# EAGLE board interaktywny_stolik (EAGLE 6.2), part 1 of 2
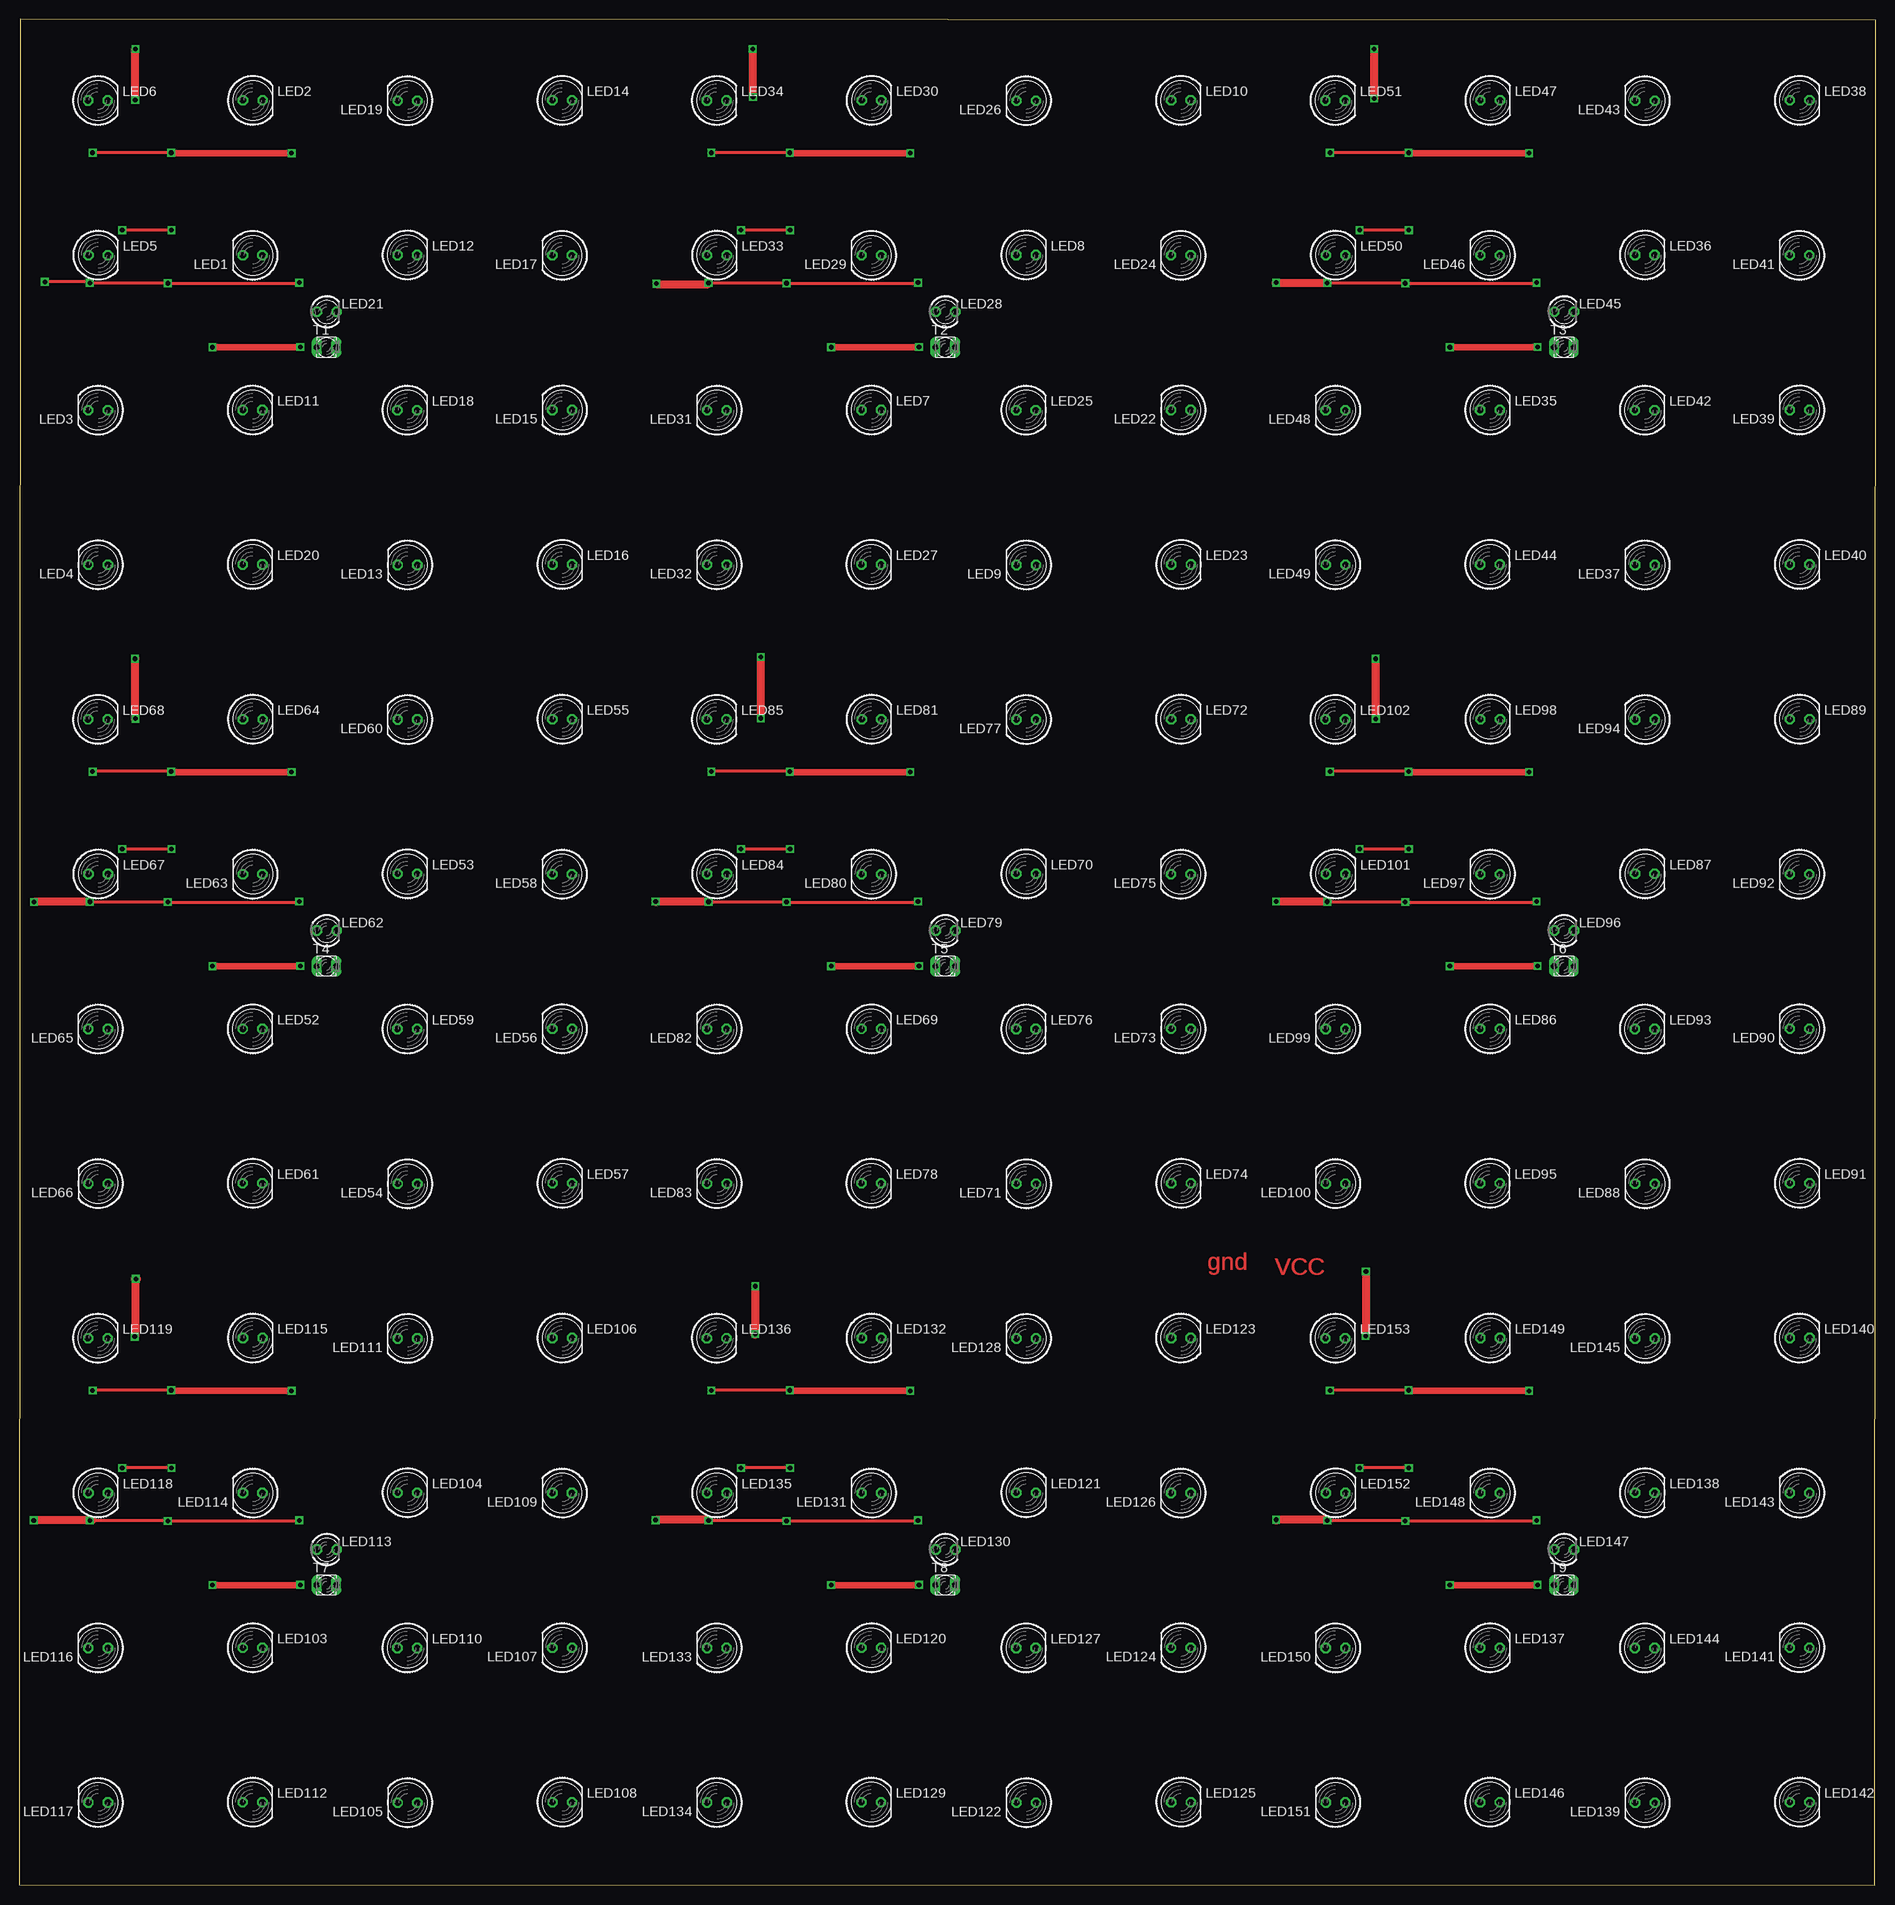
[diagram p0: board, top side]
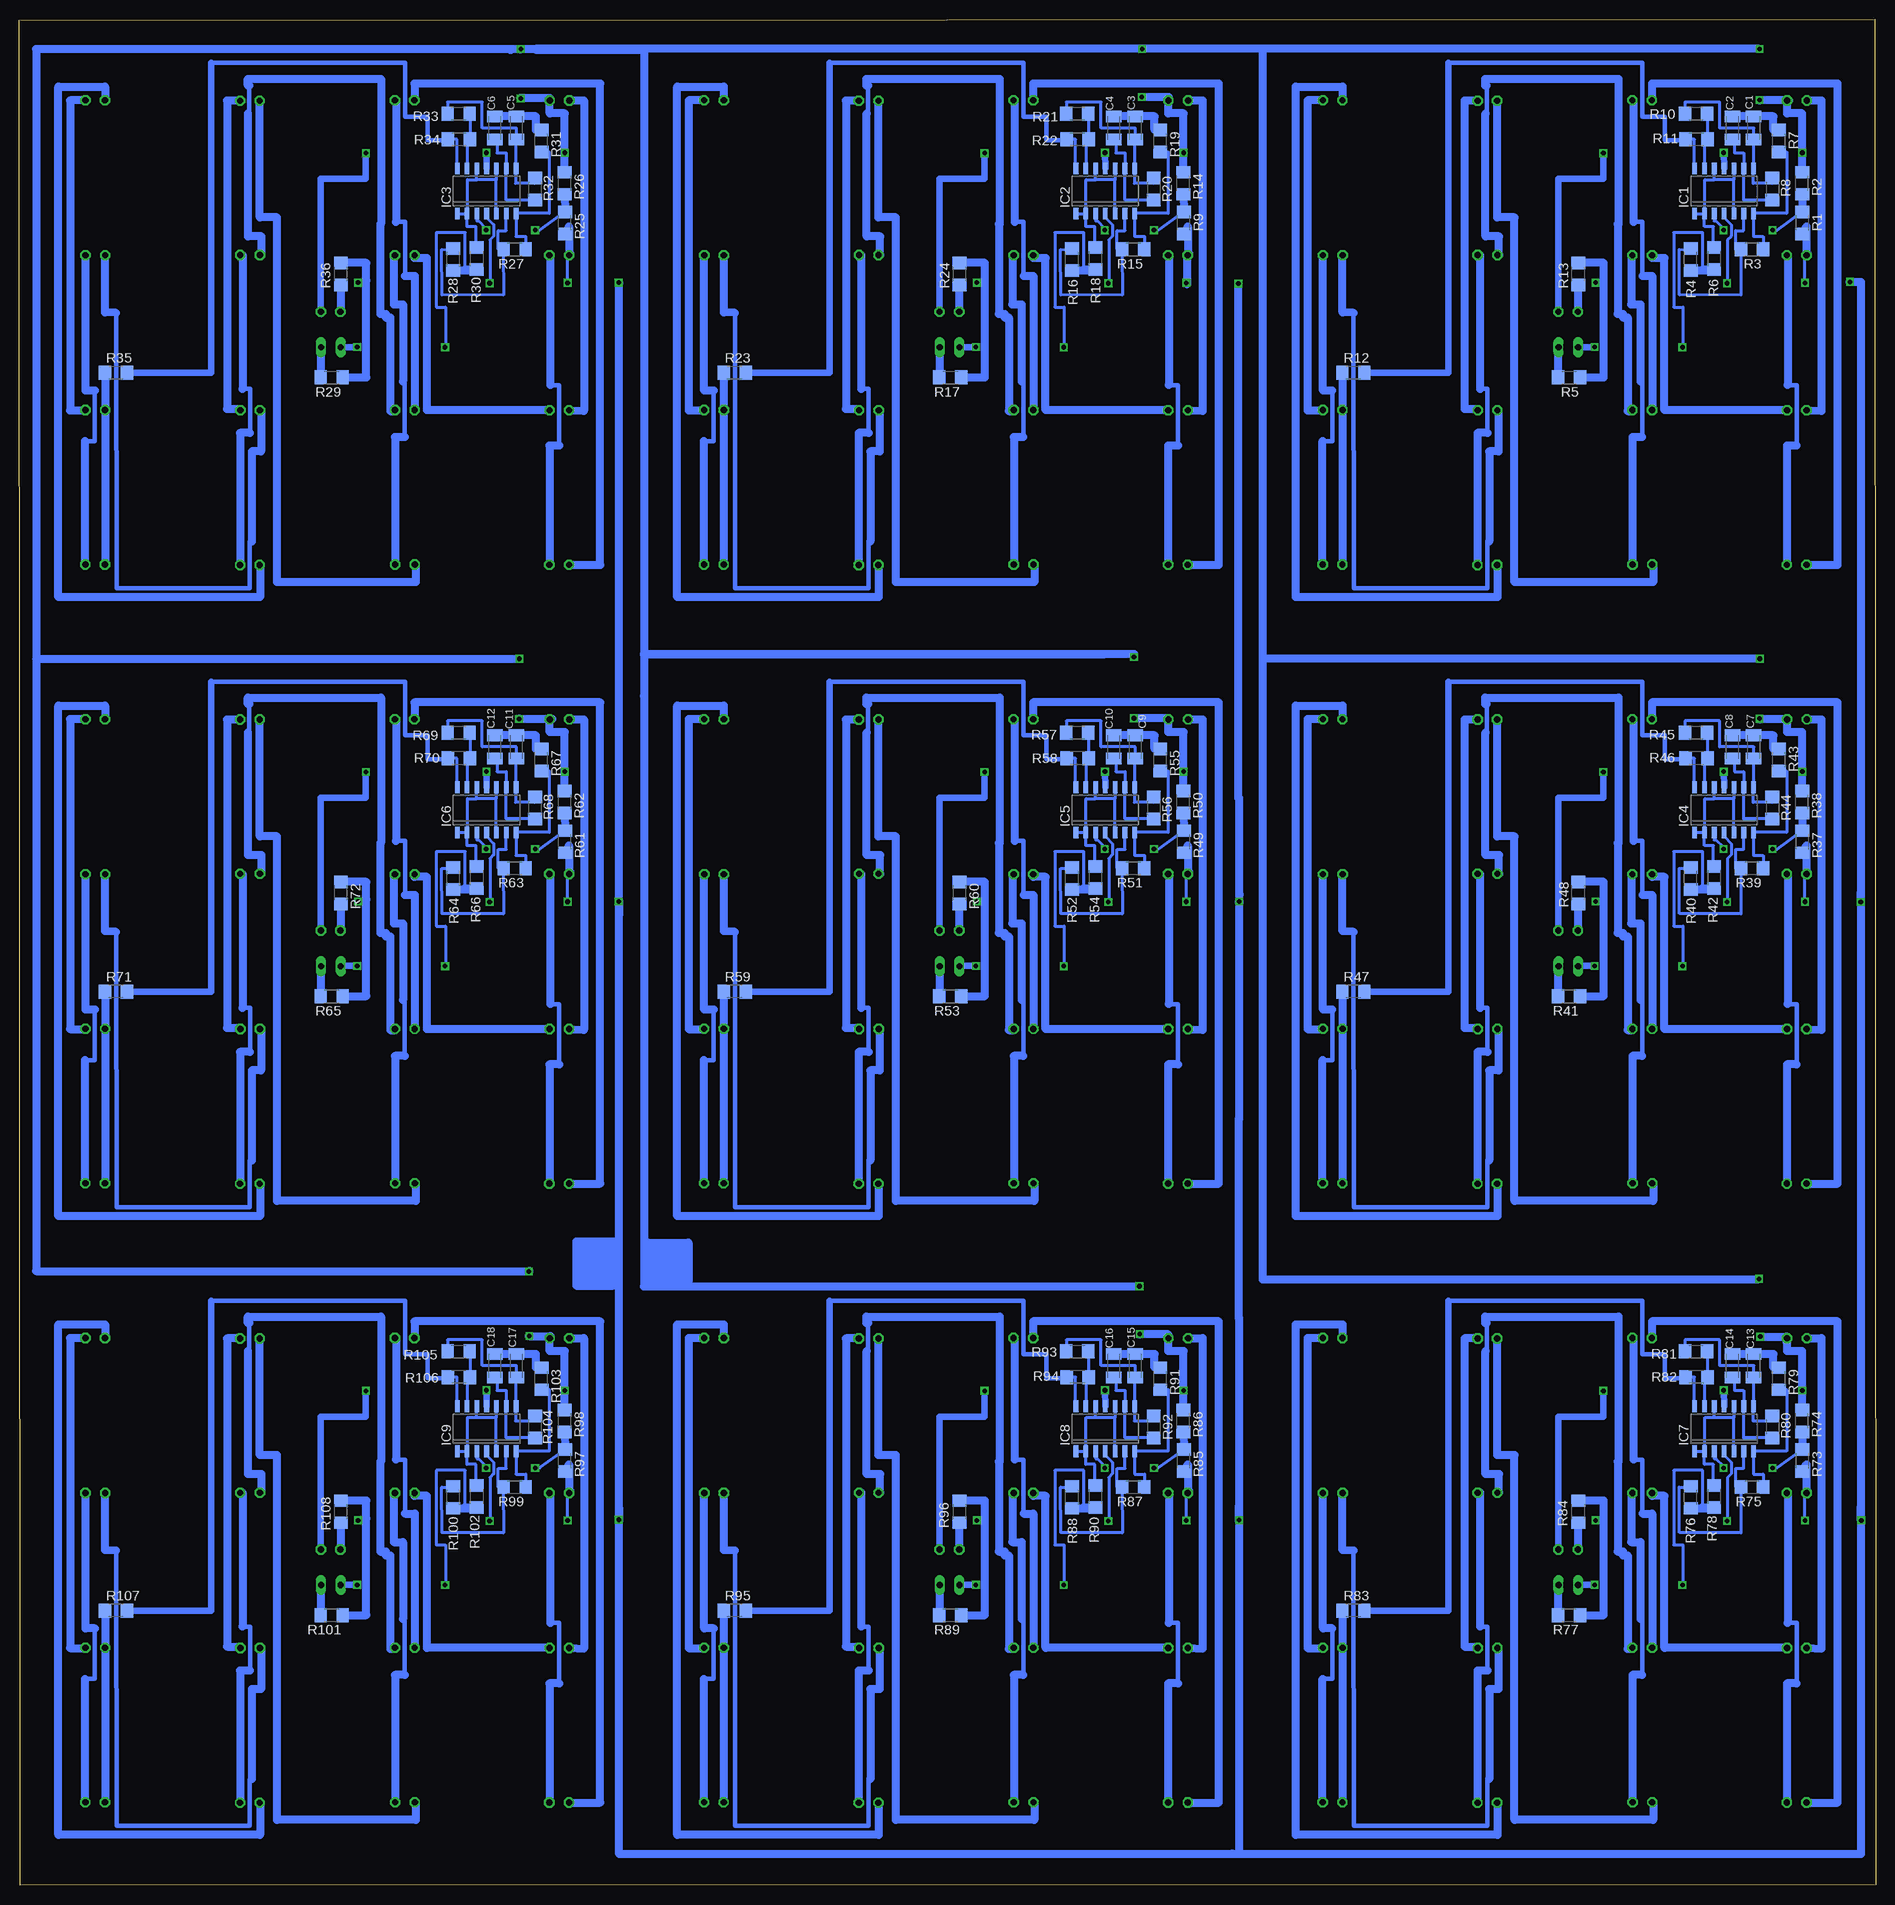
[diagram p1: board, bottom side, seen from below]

Size 240.01 x 241.21 mm. Coordinates in mm from the lower left corner, seen from the top.
Outline: 0,0.1 239.91,0 240.01,241.11 0.1,241.21 0,0.1
Copper layers (1*16): Top 0.035mm / dielectric 1.5mm / Bottom 0.035mm
Design rules: minimum track width 10mil, minimum drill 24mil, track to track 8mil, track to pad 8mil, pad to pad 8mil, via to via 8mil, smd to smd 8mil, copper to edge 40mil, drill to drill 8mil, minimum pad ring 10mil, minimum via ring 8mil, stop-mask expansion 4mil, vias tented up to drill 0mil, thermal gap 10mil

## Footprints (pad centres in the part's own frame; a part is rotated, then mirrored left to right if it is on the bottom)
C1206K = smd 1.5 x 2: 1 -1.5,0; 2 1.5,0
SO14 = smd 0.6 x 1.524: 1 -3.81,-2.935; 2 -2.54,-2.935; 3 -1.27,-2.935; 4 0,-2.935; 5 1.27,-2.935; 6 2.54,-2.935; 7 3.81,-2.935; 8 3.81,2.9; 9 2.54,2.9; 10 1.27,2.9; 11 0,2.9; 12 -1.27,2.9; 13 -2.54,2.9; 14 -3.81,2.9
LED5MM = drill 0.813 octagon: A -1.27,0; K 1.27,0
LED3MM = drill 0.813 octagon: A -1.27,0; K 1.27,0
R1206 = smd 1.6 x 1.803: 1 -1.422,0; 2 1.422,0
BPX81 = drill 0.813 long: C 1.27,0; E -1.27,0

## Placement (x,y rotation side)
C1  [C1206K]  15.75,227.16 270 bottom
C2  [C1206K]  18.52,227.16 270 bottom
C3  [C1206K]  95.75,227.16 270 bottom
C4  [C1206K]  98.52,227.16 270 bottom
C5  [C1206K]  175.75,227.16 270 bottom
C6  [C1206K]  178.52,227.16 270 bottom
C7  [C1206K]  15.75,147.16 270 bottom
C8  [C1206K]  18.52,147.16 270 bottom
C9  [C1206K]  95.75,147.16 270 bottom
C10  [C1206K]  98.52,147.16 270 bottom
C11  [C1206K]  175.75,147.16 270 bottom
C12  [C1206K]  178.52,147.16 270 bottom
C13  [C1206K]  15.75,67.16 270 bottom
C14  [C1206K]  18.52,67.16 270 bottom
C15  [C1206K]  95.75,67.16 270 bottom
C16  [C1206K]  98.52,67.16 270 bottom
C17  [C1206K]  175.75,67.16 270 bottom
C18  [C1206K]  178.52,67.16 270 bottom
IC1  LM324D  [SO14]  19.58,219.03 0 bottom
IC2  LM324D  [SO14]  99.58,219.03 0 bottom
IC3  LM324D  [SO14]  179.58,219.03 0 bottom
IC4  LM324D  [SO14]  19.58,139.03 0 bottom
IC5  LM324D  [SO14]  99.58,139.03 0 bottom
IC6  LM324D  [SO14]  179.58,139.03 0 bottom
IC7  LM324D  [SO14]  19.58,59.03 0 bottom
IC8  LM324D  [SO14]  99.58,59.03 0 bottom
IC9  LM324D  [SO14]  179.58,59.03 0 bottom
LED1  [LED5MM]  30.18,210.7 180 top
LED2  [LED5MM]  30.19,230.74 0 top
LED3  [LED5MM]  10.19,190.69 180 top
LED4  [LED5MM]  10.2,170.7 180 top
LED5  [LED5MM]  10.2,210.72 0 top
LED6  [LED5MM]  10.16,230.72 0 top
LED7  [LED5MM]  110.16,190.71 0 top
LED8  [LED5MM]  130.18,210.75 0 top
LED9  [LED5MM]  130.2,170.68 180 top
LED10  [LED5MM]  150.2,230.74 0 top
LED11  [LED5MM]  30.16,190.71 0 top
LED12  [LED5MM]  50.18,210.75 0 top
LED13  [LED5MM]  50.2,170.68 180 top
LED14  [LED5MM]  70.2,230.74 0 top
LED15  [LED5MM]  70.19,190.72 180 top
LED16  [LED5MM]  70.21,170.75 0 top
LED17  [LED5MM]  70.18,210.7 180 top
LED18  [LED5MM]  50.16,190.69 0 top
LED19  [LED5MM]  50.19,230.69 180 top
LED20  [LED5MM]  30.15,170.75 0 top
LED21  [LED3MM]  39.75,203.41 0 top
LED22  [LED5MM]  150.19,190.72 180 top
LED23  [LED5MM]  150.21,170.75 0 top
LED24  [LED5MM]  150.18,210.7 180 top
LED25  [LED5MM]  130.16,190.69 0 top
LED26  [LED5MM]  130.19,230.69 180 top
LED27  [LED5MM]  110.15,170.75 0 top
LED28  [LED3MM]  119.75,203.41 0 top
LED29  [LED5MM]  110.18,210.7 180 top
LED30  [LED5MM]  110.19,230.74 0 top
LED31  [LED5MM]  90.19,190.69 180 top
LED32  [LED5MM]  90.2,170.7 180 top
LED33  [LED5MM]  90.2,210.72 0 top
LED34  [LED5MM]  90.16,230.72 0 top
LED35  [LED5MM]  190.16,190.71 0 top
LED36  [LED5MM]  210.18,210.75 0 top
LED37  [LED5MM]  210.2,170.68 180 top
LED38  [LED5MM]  230.2,230.74 0 top
LED39  [LED5MM]  230.19,190.72 180 top
LED40  [LED5MM]  230.21,170.75 0 top
LED41  [LED5MM]  230.18,210.7 180 top
LED42  [LED5MM]  210.16,190.69 0 top
LED43  [LED5MM]  210.19,230.69 180 top
LED44  [LED5MM]  190.15,170.75 0 top
LED45  [LED3MM]  199.75,203.41 0 top
LED46  [LED5MM]  190.18,210.7 180 top
LED47  [LED5MM]  190.19,230.74 0 top
LED48  [LED5MM]  170.19,190.69 180 top
LED49  [LED5MM]  170.2,170.7 180 top
LED50  [LED5MM]  170.2,210.72 0 top
LED51  [LED5MM]  170.16,230.72 0 top
LED52  [LED5MM]  30.16,110.71 0 top
LED53  [LED5MM]  50.18,130.75 0 top
LED54  [LED5MM]  50.2,90.68 180 top
LED55  [LED5MM]  70.2,150.74 0 top
LED56  [LED5MM]  70.19,110.72 180 top
LED57  [LED5MM]  70.21,90.75 0 top
LED58  [LED5MM]  70.18,130.7 180 top
LED59  [LED5MM]  50.16,110.69 0 top
LED60  [LED5MM]  50.19,150.69 180 top
LED61  [LED5MM]  30.15,90.75 0 top
LED62  [LED3MM]  39.75,123.41 0 top
LED63  [LED5MM]  30.18,130.7 180 top
LED64  [LED5MM]  30.19,150.74 0 top
LED65  [LED5MM]  10.19,110.69 180 top
LED66  [LED5MM]  10.2,90.7 180 top
LED67  [LED5MM]  10.2,130.72 0 top
LED68  [LED5MM]  10.16,150.72 0 top
LED69  [LED5MM]  110.16,110.71 0 top
LED70  [LED5MM]  130.18,130.75 0 top
LED71  [LED5MM]  130.2,90.68 180 top
LED72  [LED5MM]  150.2,150.74 0 top
LED73  [LED5MM]  150.19,110.72 180 top
LED74  [LED5MM]  150.21,90.75 0 top
LED75  [LED5MM]  150.18,130.7 180 top
LED76  [LED5MM]  130.16,110.69 0 top
LED77  [LED5MM]  130.19,150.69 180 top
LED78  [LED5MM]  110.15,90.75 0 top
LED79  [LED3MM]  119.75,123.41 0 top
LED80  [LED5MM]  110.18,130.7 180 top
LED81  [LED5MM]  110.19,150.74 0 top
LED82  [LED5MM]  90.19,110.69 180 top
LED83  [LED5MM]  90.2,90.7 180 top
LED84  [LED5MM]  90.2,130.72 0 top
LED85  [LED5MM]  90.16,150.72 0 top
LED86  [LED5MM]  190.16,110.71 0 top
LED87  [LED5MM]  210.18,130.75 0 top
LED88  [LED5MM]  210.2,90.68 180 top
LED89  [LED5MM]  230.2,150.74 0 top
LED90  [LED5MM]  230.19,110.72 180 top
LED91  [LED5MM]  230.21,90.75 0 top
LED92  [LED5MM]  230.18,130.7 180 top
LED93  [LED5MM]  210.16,110.69 0 top
LED94  [LED5MM]  210.19,150.69 180 top
LED95  [LED5MM]  190.15,90.75 0 top
LED96  [LED3MM]  199.75,123.41 0 top
LED97  [LED5MM]  190.18,130.7 180 top
LED98  [LED5MM]  190.19,150.74 0 top
LED99  [LED5MM]  170.19,110.69 180 top
LED100  [LED5MM]  170.2,90.7 180 top
LED101  [LED5MM]  170.2,130.72 0 top
LED102  [LED5MM]  170.16,150.72 0 top
LED103  [LED5MM]  30.16,30.71 0 top
LED104  [LED5MM]  50.18,50.75 0 top
LED105  [LED5MM]  50.2,10.68 180 top
LED106  [LED5MM]  70.2,70.74 0 top
LED107  [LED5MM]  70.19,30.72 180 top
LED108  [LED5MM]  70.21,10.75 0 top
LED109  [LED5MM]  70.18,50.7 180 top
LED110  [LED5MM]  50.16,30.69 0 top
LED111  [LED5MM]  50.19,70.69 180 top
LED112  [LED5MM]  30.15,10.75 0 top
LED113  [LED3MM]  39.75,43.41 0 top
LED114  [LED5MM]  30.18,50.7 180 top
LED115  [LED5MM]  30.19,70.74 0 top
LED116  [LED5MM]  10.19,30.69 180 top
LED117  [LED5MM]  10.2,10.7 180 top
LED118  [LED5MM]  10.2,50.72 0 top
LED119  [LED5MM]  10.16,70.72 0 top
LED120  [LED5MM]  110.16,30.71 0 top
LED121  [LED5MM]  130.18,50.75 0 top
LED122  [LED5MM]  130.2,10.68 180 top
LED123  [LED5MM]  150.2,70.74 0 top
LED124  [LED5MM]  150.19,30.72 180 top
LED125  [LED5MM]  150.21,10.75 0 top
LED126  [LED5MM]  150.18,50.7 180 top
LED127  [LED5MM]  130.16,30.69 0 top
LED128  [LED5MM]  130.19,70.69 180 top
LED129  [LED5MM]  110.15,10.75 0 top
LED130  [LED3MM]  119.75,43.41 0 top
LED131  [LED5MM]  110.18,50.7 180 top
LED132  [LED5MM]  110.19,70.74 0 top
LED133  [LED5MM]  90.19,30.69 180 top
LED134  [LED5MM]  90.2,10.7 180 top
LED135  [LED5MM]  90.2,50.72 0 top
LED136  [LED5MM]  90.16,70.72 0 top
LED137  [LED5MM]  190.16,30.71 0 top
LED138  [LED5MM]  210.18,50.75 0 top
LED139  [LED5MM]  210.2,10.68 180 top
LED140  [LED5MM]  230.2,70.74 0 top
LED141  [LED5MM]  230.19,30.72 180 top
LED142  [LED5MM]  230.21,10.75 0 top
LED143  [LED5MM]  230.18,50.7 180 top
LED144  [LED5MM]  210.16,30.69 0 top
LED145  [LED5MM]  210.19,70.69 180 top
LED146  [LED5MM]  190.15,10.75 0 top
LED147  [LED3MM]  199.75,43.41 0 top
LED148  [LED5MM]  190.18,50.7 180 top
LED149  [LED5MM]  190.19,70.74 0 top
LED150  [LED5MM]  170.19,30.69 180 top
LED151  [LED5MM]  170.2,10.7 180 top
LED152  [LED5MM]  170.2,50.72 0 top
LED153  [LED5MM]  170.16,70.72 0 top
R1  [R1206]  9.45,214.89 270 bottom
R2  [R1206]  9.5,220.03 270 bottom
R3  [R1206]  15.98,211.49 180 bottom
R4  [R1206]  23.9,210.17 270 bottom
R5  [R1206]  39.62,194.93 180 bottom
R6  [R1206]  20.88,210.27 90 bottom
R7  [R1206]  12.5,225.49 270 bottom
R8  [R1206]  13.33,219.26 90 bottom
R9  [R1206]  89.45,214.89 270 bottom
R10  [R1206]  23.22,229.02 180 bottom
R11  [R1206]  23.16,225.69 0 bottom
R12  [R1206]  67.51,195.51 0 bottom
R13  [R1206]  38.43,208.29 270 bottom
R14  [R1206]  89.5,220.03 270 bottom
R15  [R1206]  95.98,211.49 180 bottom
R16  [R1206]  103.9,210.17 270 bottom
R17  [R1206]  119.62,194.93 180 bottom
R18  [R1206]  100.88,210.27 90 bottom
R19  [R1206]  92.5,225.49 270 bottom
R20  [R1206]  93.33,219.26 90 bottom
R21  [R1206]  103.22,229.02 180 bottom
R22  [R1206]  103.16,225.69 0 bottom
R23  [R1206]  147.51,195.51 0 bottom
R24  [R1206]  118.43,208.29 270 bottom
R25  [R1206]  169.45,214.89 270 bottom
R26  [R1206]  169.5,220.03 270 bottom
R27  [R1206]  175.98,211.49 180 bottom
R28  [R1206]  183.9,210.17 270 bottom
R29  [R1206]  199.62,194.93 180 bottom
R30  [R1206]  180.88,210.27 90 bottom
R31  [R1206]  172.5,225.49 270 bottom
R32  [R1206]  173.34,219.26 90 bottom
R33  [R1206]  183.22,229.02 180 bottom
R34  [R1206]  183.16,225.69 0 bottom
R35  [R1206]  227.51,195.51 0 bottom
R36  [R1206]  198.43,208.29 270 bottom
R37  [R1206]  9.45,134.89 270 bottom
R38  [R1206]  9.5,140.03 270 bottom
R39  [R1206]  15.98,131.49 180 bottom
R40  [R1206]  23.9,130.17 270 bottom
R41  [R1206]  39.62,114.93 180 bottom
R42  [R1206]  20.88,130.27 90 bottom
R43  [R1206]  12.5,145.49 270 bottom
R44  [R1206]  13.33,139.26 90 bottom
R45  [R1206]  23.22,149.02 180 bottom
R46  [R1206]  23.16,145.69 0 bottom
R47  [R1206]  67.51,115.51 0 bottom
R48  [R1206]  38.43,128.29 270 bottom
R49  [R1206]  89.45,134.89 270 bottom
R50  [R1206]  89.5,140.03 270 bottom
R51  [R1206]  95.98,131.49 180 bottom
R52  [R1206]  103.9,130.17 270 bottom
R53  [R1206]  119.62,114.93 180 bottom
R54  [R1206]  100.88,130.27 90 bottom
R55  [R1206]  92.5,145.49 270 bottom
R56  [R1206]  93.33,139.26 90 bottom
R57  [R1206]  103.22,149.02 180 bottom
R58  [R1206]  103.16,145.69 0 bottom
R59  [R1206]  147.51,115.51 0 bottom
R60  [R1206]  118.43,128.29 270 bottom
R61  [R1206]  169.45,134.89 270 bottom
R62  [R1206]  169.5,140.03 270 bottom
R63  [R1206]  175.98,131.49 180 bottom
R64  [R1206]  183.9,130.17 270 bottom
R65  [R1206]  199.62,114.93 180 bottom
R66  [R1206]  180.88,130.27 90 bottom
R67  [R1206]  172.5,145.49 270 bottom
R68  [R1206]  173.34,139.26 90 bottom
R69  [R1206]  183.22,149.02 180 bottom
R70  [R1206]  183.16,145.69 0 bottom
R71  [R1206]  227.51,115.51 0 bottom
R72  [R1206]  198.43,128.29 270 bottom
R73  [R1206]  9.45,54.89 270 bottom
R74  [R1206]  9.5,60.03 270 bottom
R75  [R1206]  15.98,51.49 180 bottom
R76  [R1206]  23.9,50.17 270 bottom
R77  [R1206]  39.62,34.93 180 bottom
R78  [R1206]  20.88,50.27 90 bottom
R79  [R1206]  12.5,65.49 270 bottom
R80  [R1206]  13.33,59.26 90 bottom
R81  [R1206]  23.22,69.02 180 bottom
R82  [R1206]  23.16,65.69 0 bottom
R83  [R1206]  67.51,35.51 0 bottom
R84  [R1206]  38.43,48.29 270 bottom
R85  [R1206]  89.45,54.89 270 bottom
R86  [R1206]  89.5,60.03 270 bottom
R87  [R1206]  95.98,51.49 180 bottom
R88  [R1206]  103.9,50.17 270 bottom
R89  [R1206]  119.62,34.93 180 bottom
R90  [R1206]  100.88,50.27 90 bottom
R91  [R1206]  92.5,65.49 270 bottom
R92  [R1206]  93.33,59.26 90 bottom
R93  [R1206]  103.22,69.02 180 bottom
R94  [R1206]  103.16,65.69 0 bottom
R95  [R1206]  147.51,35.51 0 bottom
R96  [R1206]  118.43,48.29 270 bottom
R97  [R1206]  169.45,54.89 270 bottom
R98  [R1206]  169.5,60.03 270 bottom
R99  [R1206]  175.98,51.49 180 bottom
R100  [R1206]  183.9,50.17 270 bottom
R101  [R1206]  199.62,34.93 180 bottom
R102  [R1206]  180.88,50.27 90 bottom
R103  [R1206]  172.5,65.49 270 bottom
R104  [R1206]  173.34,59.26 90 bottom
R105  [R1206]  183.22,69.02 180 bottom
R106  [R1206]  183.16,65.69 0 bottom
R107  [R1206]  227.51,35.51 0 bottom
R108  [R1206]  198.43,48.29 270 bottom
T1  BPX81  [BPX81]  39.73,198.82 0 top
T2  BPX81  [BPX81]  119.73,198.82 0 top
T3  BPX81  [BPX81]  199.73,198.82 0 top
T4  BPX81  [BPX81]  39.73,118.82 0 top
T5  BPX81  [BPX81]  119.73,118.82 0 top
T6  BPX81  [BPX81]  199.73,118.82 0 top
T7  BPX81  [BPX81]  39.73,38.82 0 top
T8  BPX81  [BPX81]  119.73,38.82 0 top
T9  BPX81  [BPX81]  199.73,38.82 0 top

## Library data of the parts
C1-C18 R1-R108 = rcl
IC1-IC9 = linear
LED1-LED153 = led
T1-T9 = opto-trans-siemens; OC_FARNELL: unknown; OC_NEWARK: unknown

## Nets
0V: IC1.1 IC1.2 IC1.5 IC1.10 IC1.12 R6.2
0V1: IC2.1 IC2.2 IC2.5 IC2.10 IC2.12 R18.2
0V2: IC3.1 IC3.2 IC3.5 IC3.10 IC3.12 R30.2
0V3: IC4.1 IC4.2 IC4.5 IC4.10 IC4.12 R42.2
0V4: IC5.1 IC5.2 IC5.5 IC5.10 IC5.12 R54.2
0V5: IC6.1 IC6.2 IC6.5 IC6.10 IC6.12 R66.2
0V6: IC7.1 IC7.2 IC7.5 IC7.10 IC7.12 R78.2
0V7: IC8.1 IC8.2 IC8.5 IC8.10 IC8.12 R90.2
0V8: IC9.1 IC9.2 IC9.5 IC9.10 IC9.12 R102.2
GND: IC1.11 LED6.K LED21.K R2.1
GND1: IC2.11 LED28.K LED34.K R14.1
GND2: IC3.11 LED45.K LED51.K R26.1
GND3: IC4.11 LED62.K LED68.K R38.1
GND4: IC5.11 LED79.K LED85.K R50.1
GND5: IC6.11 LED96.K LED102.K R62.1
GND6: IC7.11 LED113.K LED119.K R74.1
GND7: IC8.11 LED130.K LED136.K R86.1
GND8: IC9.11 LED147.K LED153.K R98.1
N$1: IC1.3 R1.1 R2.2
N$2: IC1.6 R3.2 R4.1
N$3: IC1.7 R3.1 R7.2
N$4: R4.2 R6.1 T1.E
N$5: R5.2 T1.C
N$6: C2.2 IC1.9 R8.1
N$7: C1.2 IC1.8 R8.2 R10.2
N$8: IC1.13 R10.1 R11.2
N$9: C1.1 C2.1 R7.1
N$10: IC1.14 R11.1 R12.2
N$11: LED1.A LED20.K
N$12: LED2.K LED11.A
N$13: LED1.K LED3.A
N$14: LED2.A LED4.K
N$15: LED4.A LED5.K
N$16: LED3.K LED6.A
N$17: LED21.A R13.2
N$18: IC2.3 R9.1 R14.2
N$19: IC2.6 R15.2 R16.1
N$20: IC2.7 R15.1 R19.2
N$21: R16.2 R18.1 T2.E
N$22: LED11.K LED12.A
N$23: LED12.K LED13.A
N$24: LED13.K LED14.A
N$25: LED14.K LED15.A
N$26: LED15.K LED16.A R12.1
N$27: LED16.K LED17.A
N$28: LED17.K LED18.A
N$29: LED18.K LED19.A
N$30: LED19.K LED20.A
N$31: R17.2 T2.C
N$32: C4.2 IC2.9 R20.1
N$33: C3.2 IC2.8 R20.2 R21.2
N$34: C3.1 C4.1 R19.1
N$35: IC2.13 R21.1 R22.2
N$36: IC2.14 R22.1 R23.2
N$37: LED7.K LED8.A
N$38: LED8.K LED9.A
N$39: LED9.K LED10.A
N$40: LED10.K LED22.A
N$41: LED22.K LED23.A R23.1
N$42: LED23.K LED24.A
N$43: LED24.K LED25.A
N$44: LED25.K LED26.A
N$45: LED26.K LED27.A
N$46: LED27.K LED29.A
N$47: LED7.A LED30.K
N$48: LED29.K LED31.A
N$49: LED30.A LED32.K
N$50: LED32.A LED33.K
N$51: LED31.K LED34.A
N$52: LED28.A R24.2
N$53: IC3.3 R25.1 R26.2
N$54: IC3.6 R27.2 R28.1
N$55: IC3.7 R27.1 R31.2
N$56: R28.2 R30.1 T3.E
N$57: R29.2 T3.C
N$58: C6.2 IC3.9 R32.1
N$59: C5.2 IC3.8 R32.2 R33.2
N$60: C5.1 C6.1 R31.1
N$61: IC3.13 R33.1 R34.2
N$62: IC3.14 R34.1 R35.2
N$63: LED35.K LED36.A
N$64: LED36.K LED37.A
N$65: LED37.K LED38.A
N$66: LED38.K LED39.A
N$67: LED39.K LED40.A R35.1
N$68: LED40.K LED41.A
N$69: LED41.K LED42.A
N$70: LED42.K LED43.A
N$71: LED43.K LED44.A
N$72: LED44.K LED46.A
N$73: LED35.A LED47.K
N$74: LED46.K LED48.A
N$75: LED47.A LED49.K
N$76: LED49.A LED50.K
N$77: LED48.K LED51.A
N$78: LED45.A R36.2
N$79: IC4.3 R37.1 R38.2
N$80: IC4.6 R39.2 R40.1
N$81: IC4.7 R39.1 R43.2
N$82: R40.2 R42.1 T4.E
N$83: R41.2 T4.C
N$84: C8.2 IC4.9 R44.1
N$85: C7.2 IC4.8 R44.2 R45.2
N$86: C7.1 C8.1 R43.1
N$87: IC4.13 R45.1 R46.2
N$88: IC4.14 R46.1 R47.2
N$89: LED52.K LED53.A
N$90: LED53.K LED54.A
N$91: LED54.K LED55.A
N$92: LED55.K LED56.A
N$93: LED56.K LED57.A R47.1
N$94: LED57.K LED58.A
N$95: LED58.K LED59.A
N$96: LED59.K LED60.A
N$97: LED60.K LED61.A
N$98: LED61.K LED63.A
N$99: LED52.A LED64.K
N$100: LED63.K LED65.A
N$101: LED64.A LED66.K
N$102: LED66.A LED67.K
N$103: LED65.K LED68.A
N$104: LED62.A R48.2
N$105: IC5.3 R49.1 R50.2
N$106: IC5.6 R51.2 R52.1
N$107: IC5.7 R51.1 R55.2
N$108: R52.2 R54.1 T5.E
N$109: R53.2 T5.C
N$110: C10.2 IC5.9 R56.1
N$111: C9.2 IC5.8 R56.2 R57.2
N$112: C9.1 C10.1 R55.1
N$113: IC5.13 R57.1 R58.2
N$114: IC5.14 R58.1 R59.2
N$115: LED69.K LED70.A
N$116: LED70.K LED71.A
N$117: LED71.K LED72.A
N$118: LED72.K LED73.A
N$119: LED73.K LED74.A R59.1
N$120: LED74.K LED75.A
N$121: LED75.K LED76.A
N$122: LED76.K LED77.A
N$123: LED77.K LED78.A
N$124: LED78.K LED80.A
N$125: LED69.A LED81.K
N$126: LED80.K LED82.A
N$127: LED81.A LED83.K
N$128: LED83.A LED84.K
N$129: LED82.K LED85.A
N$130: LED79.A R60.2
N$131: IC6.3 R61.1 R62.2
N$132: IC6.6 R63.2 R64.1
N$133: IC6.7 R63.1 R67.2
N$134: R64.2 R66.1 T6.E
N$135: R65.2 T6.C
N$136: C12.2 IC6.9 R68.1
N$137: C11.2 IC6.8 R68.2 R69.2
N$138: C11.1 C12.1 R67.1
N$139: IC6.13 R69.1 R70.2
N$140: IC6.14 R70.1 R71.2
N$141: LED86.K LED87.A
N$142: LED87.K LED88.A
N$143: LED88.K LED89.A
N$144: LED89.K LED90.A
N$145: LED90.K LED91.A R71.1
N$146: LED91.K LED92.A
N$147: LED92.K LED93.A
N$148: LED93.K LED94.A
N$149: LED94.K LED95.A
N$150: LED95.K LED97.A
N$151: LED86.A LED98.K
N$152: LED97.K LED99.A
N$153: LED98.A LED100.K
N$154: LED100.A LED101.K
N$155: LED99.K LED102.A
N$156: LED96.A R72.2
N$157: IC7.3 R73.1 R74.2
N$158: IC7.6 R75.2 R76.1
N$159: IC7.7 R75.1 R79.2
N$160: R76.2 R78.1 T7.E
N$161: R77.2 T7.C
N$162: C14.2 IC7.9 R80.1
N$163: C13.2 IC7.8 R80.2 R81.2
N$164: C13.1 C14.1 R79.1
N$165: IC7.13 R81.1 R82.2
N$166: IC7.14 R82.1 R83.2
N$167: LED103.K LED104.A
N$168: LED104.K LED105.A
N$169: LED105.K LED106.A
N$170: LED106.K LED107.A
N$171: LED107.K LED108.A R83.1
N$172: LED108.K LED109.A
N$173: LED109.K LED110.A
N$174: LED110.K LED111.A
N$175: LED111.K LED112.A
N$176: LED112.K LED114.A
N$177: LED103.A LED115.K
N$178: LED114.K LED116.A
N$179: LED115.A LED117.K
N$180: LED117.A LED118.K
N$181: LED116.K LED119.A
N$182: LED113.A R84.2
N$183: IC8.3 R85.1 R86.2
N$184: IC8.6 R87.2 R88.1
N$185: IC8.7 R87.1 R91.2
N$186: R88.2 R90.1 T8.E
N$187: R89.2 T8.C
N$188: C16.2 IC8.9 R92.1
N$189: C15.2 IC8.8 R92.2 R93.2
N$190: C15.1 C16.1 R91.1
N$191: IC8.13 R93.1 R94.2
N$192: IC8.14 R94.1 R95.2
N$193: LED120.K LED121.A
N$194: LED121.K LED122.A
N$195: LED122.K LED123.A
N$196: LED123.K LED124.A
N$197: LED124.K LED125.A R95.1
N$198: LED125.K LED126.A
N$199: LED126.K LED127.A
N$200: LED127.K LED128.A
N$201: LED128.K LED129.A
N$202: LED129.K LED131.A
N$203: LED120.A LED132.K
N$204: LED131.K LED133.A
N$205: LED132.A LED134.K
N$206: LED134.A LED135.K
N$207: LED133.K LED136.A
N$208: LED130.A R96.2
N$209: IC9.3 R97.1 R98.2
N$210: IC9.6 R99.2 R100.1
N$211: IC9.7 R99.1 R103.2
N$212: R100.2 R102.1 T9.E
N$213: R101.2 T9.C
N$214: C18.2 IC9.9 R104.1
N$215: C17.2 IC9.8 R104.2 R105.2
N$216: C17.1 C18.1 R103.1
N$217: IC9.13 R105.1 R106.2
N$218: IC9.14 R106.1 R107.2
N$219: LED137.K LED138.A
N$220: LED138.K LED139.A
N$221: LED139.K LED140.A
N$222: LED140.K LED141.A
N$223: LED141.K LED142.A R107.1
N$224: LED142.K LED143.A
N$225: LED143.K LED144.A
N$226: LED144.K LED145.A
N$227: LED145.K LED146.A
N$228: LED146.K LED148.A
N$229: LED137.A LED149.K
N$230: LED148.K LED150.A
N$231: LED149.A LED151.K
N$232: LED151.A LED152.K
N$233: LED150.K LED153.A
N$234: LED147.A R108.2
VCC: IC1.4 LED5.A R1.2 R5.1 R13.1
VCC1: IC2.4 LED33.A R9.2 R17.1 R24.1
VCC2: IC3.4 LED50.A R25.2 R29.1 R36.1
VCC3: IC4.4 LED67.A R37.2 R41.1 R48.1
VCC4: IC5.4 LED84.A R49.2 R53.1 R60.1
VCC5: IC6.4 LED101.A R61.2 R65.1 R72.1
VCC6: IC7.4 LED118.A R73.2 R77.1 R84.1
VCC7: IC8.4 LED135.A R85.2 R89.1 R96.1
VCC8: IC9.4 LED152.A R97.2 R101.1 R108.1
